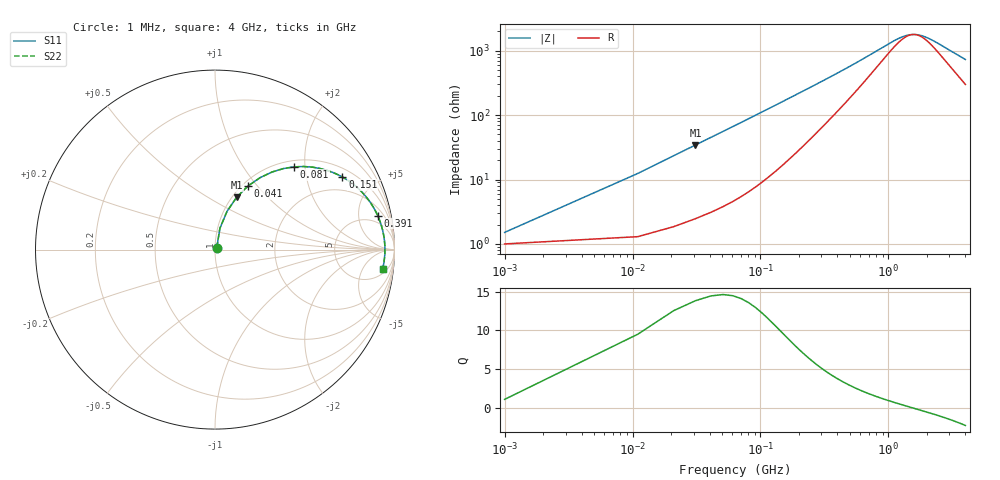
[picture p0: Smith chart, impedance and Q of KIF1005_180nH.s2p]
!version-2
!date-12.2020
!Series
# MHz S RI R 50
!Freq ReS11 ImS11 ReS21 ImS21 ReS12 ImS12 ReS22 ImS22
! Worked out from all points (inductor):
!   401 points, 1 MHz to 4 GHz, reference 50 ohm
!   read as one part in series: L = 175 nH near 21 MHz
!   highest Q = 13.8 at 31 MHz (marker M1), where L = 175 nH
!   self-resonance near 1.577 GHz
!   S11 on the Smith chart (normalised r, x): 1 MHz: 1.02, +0.02; 41 MHz: 1.06, +0.90; 81 MHz: 1.13, +1.75; 151 MHz: 1.34, +3.27; 391 MHz: 3.18, +8.47; 4 GHz: 7, -13
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1  0.01 0.0111  0.99 -0.0111  0.99 -0.0111  0.01 0.0111
11  0.0273 0.1187  0.9727 -0.1187  0.9727 -0.1187  0.0273 0.1187
31  0.1213 0.2923  0.8787 -0.2923  0.8787 -0.2923  0.1213 0.2923
41  0.1841 0.3545  0.8159 -0.3545  0.8159 -0.3545  0.1841 0.3545
51  0.2508 0.4006  0.7492 -0.4006  0.7492 -0.4006  0.2508 0.4006
61  0.3174 0.4322  0.6826 -0.4322  0.6826 -0.4322  0.3174 0.4322
81  0.4404 0.4609  0.5596 -0.4609  0.5596 -0.4609  0.4404 0.4609
111  0.5849 0.452  0.4151 -0.452  0.4151 -0.452  0.5849 0.452
151  0.7099 0.4045  0.2901 -0.4045  0.2901 -0.4045  0.7099 0.4045
191  0.7847 0.3525  0.2153 -0.3525  0.2153 -0.3525  0.7847 0.3525
241  0.8397 0.2967  0.1603 -0.2967  0.1603 -0.2967  0.8397 0.2967
391  0.9063 0.1899  0.0937 -0.1899  0.0937 -0.1899  0.9063 0.1899
521  0.9258 0.1382  0.0742 -0.1382  0.0742 -0.1382  0.9258 0.1382
671  0.936 0.0997  0.064 -0.0997  0.064 -0.0997  0.936 0.0997
1021  0.9444 0.0469  0.0556 -0.0469  0.0556 -0.0469  0.9444 0.0469
1181  0.9458 0.0307  0.0542 -0.0307  0.0542 -0.0307  0.9458 0.0307
1341  0.9465 0.0171  0.0535 -0.0171  0.0535 -0.0171  0.9465 0.0171
1631  0.9468 -0.00353  0.0532 0.00353  0.0532 0.00353  0.9468 -0.00353
2001  0.9461 -0.0252  0.0539 0.0252  0.0539 0.0252  0.9461 -0.0252
2671  0.9432 -0.0576  0.0568 0.0576  0.0568 0.0576  0.9432 -0.0576
3341  0.9389 -0.0856  0.0611 0.0856  0.0611 0.0856  0.9389 -0.0856
4000  0.9335 -0.1107  0.0665 0.1107  0.0665 0.1107  0.9335 -0.1107
